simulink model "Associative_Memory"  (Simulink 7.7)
settings: Solver=ode113  StartTime=0.0  StopTime=20  RelTol=3e-14
undefined symbols (not defined in the file or in its folder): sigbuilder_block
libraries: fl_lib x51, nesl_utility x22, Memristor_lib x2

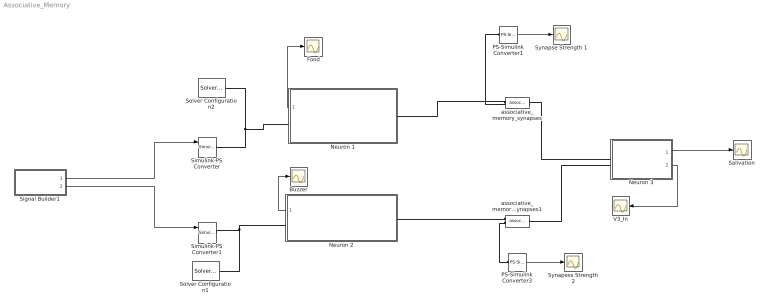
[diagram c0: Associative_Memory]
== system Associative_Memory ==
  Buzzer : Scope
  Food : Scope
  Neuron 1 : Subsystem
  Neuron 2 : Subsystem
  Neuron 3 : Subsystem
  PS-Simulink Converter1 : nesl_utility/PS-Simulink Converter  SystemSampleTime=-1  PhysicalDomain=network_engine_domain  LeftPortType=input  RightPortType=output  SubClassName=ps_output  Unit=1  AffineConversion=off
  PS-Simulink Converter3 : nesl_utility/PS-Simulink Converter  SystemSampleTime=-1  PhysicalDomain=network_engine_domain  LeftPortType=input  RightPortType=output  SubClassName=ps_output  Unit=1  AffineConversion=off
  Salivation : Scope
  Signal Builder1 : Subsystem  Tag=STV Subsys  LoadFcn=sigbuilder_block('load');  StartFcn=sigbuilder_block('start');  StopFcn=sigbuilder_block('stop');  ClipboardFcn=sigbuilder_block('clipboard');
  Simulink-PS Converter : nesl_utility/Simulink-PS Converter  SystemSampleTime=-1  PhysicalDomain=network_engine_domain  LeftPortType=input  RightPortType=output  SubClassName=ps_input  Unit=1  AffineConversion=off  InputFilterTimeConstant=.001  UdotUserProvided=2
  Simulink-PS Converter1 : nesl_utility/Simulink-PS Converter  SystemSampleTime=-1  PhysicalDomain=network_engine_domain  LeftPortType=input  RightPortType=output  SubClassName=ps_input  Unit=1  AffineConversion=off  InputFilterTimeConstant=.001  UdotUserProvided=2
  Solver Configuration1 : nesl_utility/Solver Configuration  SystemSampleTime=-1  PhysicalDomain=network_engine_domain  LeftPortType=input  RightPortType=generic  SubClassName=solver  Accelerate=off  Profile=off  ResidualTolerance=1e-9  MaxNonlinIter=3  MaxModeIter=2  DoFixedCost=off  UseLocalSampling=off  DoDC=off  LinearAlgebra=Sparse  LocalSolverSampleTime=.001  LocalSolverChoice=NE_BACKWARD_EULER_ADVANCER  UseLocalSolver=off
  Solver Configuration2 : nesl_utility/Solver Configuration  SystemSampleTime=-1  PhysicalDomain=network_engine_domain  LeftPortType=input  RightPortType=generic  SubClassName=solver  Accelerate=off  Profile=off  ResidualTolerance=1e-9  MaxNonlinIter=3  MaxModeIter=2  DoFixedCost=off  UseLocalSampling=off  DoDC=off  LinearAlgebra=Sparse  LocalSolverSampleTime=.001  LocalSolverChoice=NE_BACKWARD_EULER_ADVANCER  UseLocalSolver=off
  Synapse Strength 1 : Scope
  Synapses Strength 2 : Scope
  V3_In : Scope
  associative_memory_synapses : Memristor_lib/associative_memory_synapses  SystemSampleTime=-1  a=0 Ohm/s/V  B=15000 Ohm/s/V  VT=4 V  R1=675 Ohm  R2=1e+4 Ohm  x0=675 Ohm  i_Log=off  v_Log=off  x_Log=off  LocalVarNames=|i|v|x  LocalVarDescs=|i|v|x  LocalVarLogging=[0 0 0]
  associative_memory_synapses1 : Memristor_lib/associative_memory_synapses  SystemSampleTime=-1  a=0 Ohm/s/V  B=15000 Ohm/s/V  VT=4 V  R1=675 Ohm  R2=1e+4 Ohm  x0=1e+4 Ohm  i_Log=off  v_Log=off  x_Log=off  LocalVarNames=|i|v|x  LocalVarDescs=|i|v|x  LocalVarLogging=[0 0 0]
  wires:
  Signal Builder1/1(Food) -> Simulink-PS Converter/1
  Signal Builder1/2(Buzzer) -> Simulink-PS Converter1/1
  Neuron 3/1(Out1) -> Salivation/1
  PS-Simulink Converter3/1 -> Synapses Strength 2/1
  PS-Simulink Converter1/1 -> Synapse Strength 1/1
  Neuron 1/1(Input 1) -> Food/1
  Neuron 2/1(Input 2) -> Buzzer/1
  Neuron 3/2(V3_In) -> V3_In/1
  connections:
  Neuron 2/LConn1 -- associative_memory_synapses1/RConn1
  associative_memory_synapses/LConn1 -- Neuron 3/LConn1
  associative_memory_synapses1/LConn1 -- Neuron 3/LConn2
  PS-Simulink Converter1/LConn1 -- associative_memory_synapses/RConn2
  associative_memory_synapses/RConn1 -- Neuron 1/LConn1
  Solver Configuration2/RConn1 -- Simulink-PS Converter/RConn1 -- Neuron 1/RConn1
  Simulink-PS Converter1/RConn1 -- Neuron 2/RConn1 -- Solver Configuration1/RConn1
  associative_memory_synapses1/RConn2 -- PS-Simulink Converter3/LConn1

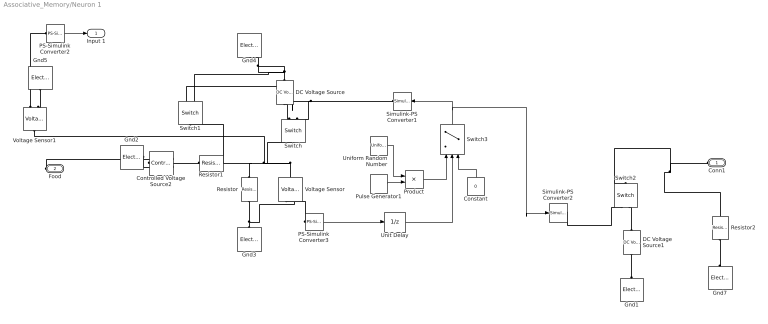
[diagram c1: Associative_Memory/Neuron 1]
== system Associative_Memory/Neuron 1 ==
  Constant : Constant  Value=0
  Controlled Voltage Source2 : fl_lib/Electrical/Electrical Sources/Controlled Voltage Source  SystemSampleTime=-1  i_Log=off  v_Log=off  LocalVarNames=|i|v  LocalVarDescs=|i|v  LocalVarLogging=[0 0]
  DC Voltage Source : fl_lib/Electrical/Electrical Sources/DC Voltage Source  SystemSampleTime=-1  v0=-2.5 V  i_Log=off  v_Log=off  LocalVarNames=|i|v  LocalVarDescs=|i|v  LocalVarLogging=[0 0]
  DC Voltage Source1 : fl_lib/Electrical/Electrical Sources/DC Voltage Source  SystemSampleTime=-1  v0=2.5 V  i_Log=off  v_Log=off  LocalVarNames=|i|v  LocalVarDescs=|i|v  LocalVarLogging=[0 0]
  Gnd{1..5,7} (6 alike) : fl_lib/Electrical/Electrical Elements/Electrical Reference  SystemSampleTime=-1  i_Log=off  LocalVarNames=|i  LocalVarDescs=|i  LocalVarLogging=0
  PS-Simulink Converter2 : nesl_utility/PS-Simulink Converter  SystemSampleTime=-1  PhysicalDomain=network_engine_domain  LeftPortType=input  RightPortType=output  SubClassName=ps_output  Unit=1  AffineConversion=off
  PS-Simulink Converter3 : nesl_utility/PS-Simulink Converter  SystemSampleTime=-1  PhysicalDomain=network_engine_domain  LeftPortType=input  RightPortType=output  SubClassName=ps_output  Unit=1  AffineConversion=off
  Product : Product  SampleTime=.001
  Pulse Generator1 : DiscretePulseGenerator  PulseType=Time based  Amplitude=1.1  Period=.1  PulseWidth=50
  Resistor : fl_lib/Electrical/Electrical Elements/Resistor  SystemSampleTime=-1  R=100 Ohm  i_Log=off  v_Log=off  LocalVarNames=|i|v  LocalVarDescs=|i|v  LocalVarLogging=[0 0]
  Resistor1 : fl_lib/Electrical/Electrical Elements/Resistor  SystemSampleTime=-1  R=50 Ohm  i_Log=off  v_Log=off  LocalVarNames=|i|v  LocalVarDescs=|i|v  LocalVarLogging=[0 0]
  Resistor2 : fl_lib/Electrical/Electrical Elements/Resistor  SystemSampleTime=-1  R=20000 Ohm  i_Log=off  v_Log=off  LocalVarNames=|i|v  LocalVarDescs=|i|v  LocalVarLogging=[0 0]
  Simulink-PS Converter1 : nesl_utility/Simulink-PS Converter  SystemSampleTime=-1  PhysicalDomain=network_engine_domain  LeftPortType=input  RightPortType=output  SubClassName=ps_input  Unit=1  AffineConversion=off  InputFilterTimeConstant=.001  UdotUserProvided=0
  Simulink-PS Converter2 : nesl_utility/Simulink-PS Converter  SystemSampleTime=-1  PhysicalDomain=network_engine_domain  LeftPortType=input  RightPortType=output  SubClassName=ps_input  Unit=1  AffineConversion=off  InputFilterTimeConstant=.001  UdotUserProvided=0
  Switch : fl_lib/Electrical/Electrical Elements/Switch  SystemSampleTime=-1  R_closed=0.01 Ohm  G_open=1e-8 1/Ohm  Threshold=.4  i_Log=off  v_Log=off  LocalVarNames=|i|v  LocalVarDescs=|i|v  LocalVarLogging=[0 0]
  Switch1 : fl_lib/Electrical/Electrical Elements/Switch  SystemSampleTime=-1  R_closed=0.01 Ohm  G_open=1e-8 1/Ohm  Threshold=1.5  i_Log=off  v_Log=off  LocalVarNames=|i|v  LocalVarDescs=|i|v  LocalVarLogging=[0 0]
  Switch2 : fl_lib/Electrical/Electrical Elements/Switch  SystemSampleTime=-1  R_closed=0.01 Ohm  G_open=1e-8 1/Ohm  Threshold=.4  i_Log=off  v_Log=off  LocalVarNames=|i|v  LocalVarDescs=|i|v  LocalVarLogging=[0 0]
  Switch3 : Switch  Threshold=1.5  SampleTime=.001
  Uniform Random Number : UniformRandomNumber  Minimum=0  Maximum=1.75  SampleTime=0.001
  Unit Delay : UnitDelay  SampleTime=.001
  Voltage Sensor : fl_lib/Electrical/Electrical Sensors/Voltage Sensor  SystemSampleTime=-1  i1_Log=off  v1_Log=off  LocalVarNames=|i1|v1  LocalVarDescs=|i1|v1  LocalVarLogging=[0 0]
  Voltage Sensor1 : fl_lib/Electrical/Electrical Sensors/Voltage Sensor  SystemSampleTime=-1  i1_Log=off  v1_Log=off  LocalVarNames=|i1|v1  LocalVarDescs=|i1|v1  LocalVarLogging=[0 0]
  Conn1 : PMIOPort  Port=1  Side=Left
  Food : PMIOPort  Port=2  Side=Right
  Input 1 : Outport
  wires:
  PS-Simulink Converter3/1 -> Unit Delay/1
  PS-Simulink Converter2/1 -> Input 1/1
  Pulse Generator1/1 -> Product/2
  Constant/1 -> Switch3/3
  Switch3/1 -> Simulink-PS Converter2/1, Simulink-PS Converter1/1
  Unit Delay/1 -> Switch3/2
  Uniform Random Number/1 -> Product/1
  Product/1 -> Switch3/1
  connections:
  Gnd2/LConn1 -- Controlled Voltage Source2/RConn2
  DC Voltage Source/LConn1 -- Switch/RConn2
  DC Voltage Source/RConn1 -- Gnd4/LConn1 -- Switch1/RConn2
  Gnd3/LConn1 -- Resistor/RConn1 -- Voltage Sensor/RConn2
  PS-Simulink Converter3/LConn1 -- Voltage Sensor/RConn1
  Voltage Sensor/LConn1 -- Switch/LConn1 -- Resistor/LConn1 -- Resistor1/LConn1 -- Voltage Sensor1/LConn1
  Simulink-PS Converter1/RConn1 -- Switch/RConn1 -- Switch1/RConn1
  Switch2/LConn1 -- Resistor2/LConn1 -- Conn1/RConn1
  Food/RConn1 -- Controlled Voltage Source2/RConn1
  Simulink-PS Converter2/RConn1 -- Switch2/RConn1
  DC Voltage Source1/LConn1 -- Switch2/RConn2
  DC Voltage Source1/RConn1 -- Gnd1/LConn1
  Gnd5/LConn1 -- Voltage Sensor1/RConn2
  Voltage Sensor1/RConn1 -- PS-Simulink Converter2/LConn1
  Resistor1/RConn1 -- Switch1/LConn1 -- Controlled Voltage Source2/LConn1
  Resistor2/RConn1 -- Gnd7/LConn1

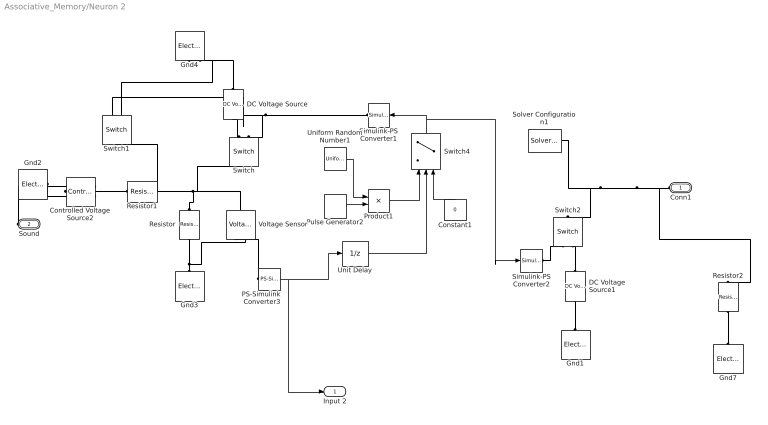
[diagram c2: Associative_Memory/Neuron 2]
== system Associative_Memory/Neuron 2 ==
  Constant1 : Constant  Value=0
  Controlled Voltage Source2 : fl_lib/Electrical/Electrical Sources/Controlled Voltage Source  SystemSampleTime=-1  i_Log=off  v_Log=off  LocalVarNames=|i|v  LocalVarDescs=|i|v  LocalVarLogging=[0 0]
  DC Voltage Source : fl_lib/Electrical/Electrical Sources/DC Voltage Source  SystemSampleTime=-1  v0=-2.5 V  i_Log=off  v_Log=off  LocalVarNames=|i|v  LocalVarDescs=|i|v  LocalVarLogging=[0 0]
  DC Voltage Source1 : fl_lib/Electrical/Electrical Sources/DC Voltage Source  SystemSampleTime=-1  v0=2.5 V  i_Log=off  v_Log=off  LocalVarNames=|i|v  LocalVarDescs=|i|v  LocalVarLogging=[0 0]
  Gnd{1..4,7} (5 alike) : fl_lib/Electrical/Electrical Elements/Electrical Reference  SystemSampleTime=-1  i_Log=off  LocalVarNames=|i  LocalVarDescs=|i  LocalVarLogging=0
  PS-Simulink Converter3 : nesl_utility/PS-Simulink Converter  SystemSampleTime=-1  PhysicalDomain=network_engine_domain  LeftPortType=input  RightPortType=output  SubClassName=ps_output  Unit=1  AffineConversion=off
  Product1 : Product  SampleTime=.001
  Pulse Generator2 : DiscretePulseGenerator  PulseType=Time based  Amplitude=1.1  Period=.1  PulseWidth=50
  Resistor : fl_lib/Electrical/Electrical Elements/Resistor  SystemSampleTime=-1  R=100 Ohm  i_Log=off  v_Log=off  LocalVarNames=|i|v  LocalVarDescs=|i|v  LocalVarLogging=[0 0]
  Resistor1 : fl_lib/Electrical/Electrical Elements/Resistor  SystemSampleTime=-1  R=50 Ohm  i_Log=off  v_Log=off  LocalVarNames=|i|v  LocalVarDescs=|i|v  LocalVarLogging=[0 0]
  Resistor2 : fl_lib/Electrical/Electrical Elements/Resistor  SystemSampleTime=-1  R=1 Ohm  i_Log=off  v_Log=off  LocalVarNames=|i|v  LocalVarDescs=|i|v  LocalVarLogging=[0 0]
  Simulink-PS Converter1 : nesl_utility/Simulink-PS Converter  SystemSampleTime=-1  PhysicalDomain=network_engine_domain  LeftPortType=input  RightPortType=output  SubClassName=ps_input  Unit=1  AffineConversion=off  InputFilterTimeConstant=.001  UdotUserProvided=0
  Simulink-PS Converter2 : nesl_utility/Simulink-PS Converter  SystemSampleTime=-1  PhysicalDomain=network_engine_domain  LeftPortType=input  RightPortType=output  SubClassName=ps_input  Unit=1  AffineConversion=off  InputFilterTimeConstant=.001  UdotUserProvided=0
  Solver Configuration1 : nesl_utility/Solver Configuration  SystemSampleTime=-1  PhysicalDomain=network_engine_domain  LeftPortType=input  RightPortType=generic  SubClassName=solver  Accelerate=off  Profile=off  ResidualTolerance=1e-9  MaxNonlinIter=3  MaxModeIter=2  DoFixedCost=off  UseLocalSampling=off  DoDC=off  LinearAlgebra=Sparse  LocalSolverSampleTime=.001  LocalSolverChoice=NE_BACKWARD_EULER_ADVANCER  UseLocalSolver=off
  Switch : fl_lib/Electrical/Electrical Elements/Switch  SystemSampleTime=-1  R_closed=0.01 Ohm  G_open=1e-8 1/Ohm  Threshold=.4  i_Log=off  v_Log=off  LocalVarNames=|i|v  LocalVarDescs=|i|v  LocalVarLogging=[0 0]
  Switch1 : fl_lib/Electrical/Electrical Elements/Switch  SystemSampleTime=-1  R_closed=0.01 Ohm  G_open=1e-8 1/Ohm  Threshold=1.5  i_Log=off  v_Log=off  LocalVarNames=|i|v  LocalVarDescs=|i|v  LocalVarLogging=[0 0]
  Switch2 : fl_lib/Electrical/Electrical Elements/Switch  SystemSampleTime=-1  R_closed=0.01 Ohm  G_open=1e-8 1/Ohm  Threshold=.4  i_Log=off  v_Log=off  LocalVarNames=|i|v  LocalVarDescs=|i|v  LocalVarLogging=[0 0]
  Switch4 : Switch  Threshold=1.5  SampleTime=.001
  Uniform Random Number1 : UniformRandomNumber  Minimum=0  Maximum=1.75  SampleTime=.001
  Unit Delay : UnitDelay  SampleTime=.001
  Voltage Sensor : fl_lib/Electrical/Electrical Sensors/Voltage Sensor  SystemSampleTime=-1  i1_Log=off  v1_Log=off  LocalVarNames=|i1|v1  LocalVarDescs=|i1|v1  LocalVarLogging=[0 0]
  Conn1 : PMIOPort  Port=1  Side=Left
  Sound : PMIOPort  Port=2  Side=Right
  Input 2 : Outport
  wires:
  PS-Simulink Converter3/1 -> Unit Delay/1, Input 2/1
  Switch4/1 -> Simulink-PS Converter1/1, Simulink-PS Converter2/1
  Pulse Generator2/1 -> Product1/2
  Constant1/1 -> Switch4/3
  Unit Delay/1 -> Switch4/2
  Uniform Random Number1/1 -> Product1/1
  Product1/1 -> Switch4/1
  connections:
  Resistor1/RConn1 -- Controlled Voltage Source2/LConn1 -- Switch1/LConn1
  Gnd2/LConn1 -- Controlled Voltage Source2/RConn2
  DC Voltage Source/LConn1 -- Switch/RConn2
  Gnd4/LConn1 -- DC Voltage Source/RConn1 -- Switch1/RConn2
  Gnd3/LConn1 -- Resistor/RConn1 -- Voltage Sensor/RConn2
  PS-Simulink Converter3/LConn1 -- Voltage Sensor/RConn1
  Resistor/LConn1 -- Voltage Sensor/LConn1 -- Switch/LConn1 -- Resistor1/LConn1
  Simulink-PS Converter1/RConn1 -- Switch/RConn1 -- Switch1/RConn1
  Conn1/RConn1 -- Switch2/LConn1 -- Solver Configuration1/RConn1 -- Resistor2/LConn1
  Sound/RConn1 -- Controlled Voltage Source2/RConn1
  DC Voltage Source1/LConn1 -- Switch2/RConn2
  DC Voltage Source1/RConn1 -- Gnd1/LConn1
  Resistor2/RConn1 -- Gnd7/LConn1
  Simulink-PS Converter2/RConn1 -- Switch2/RConn1

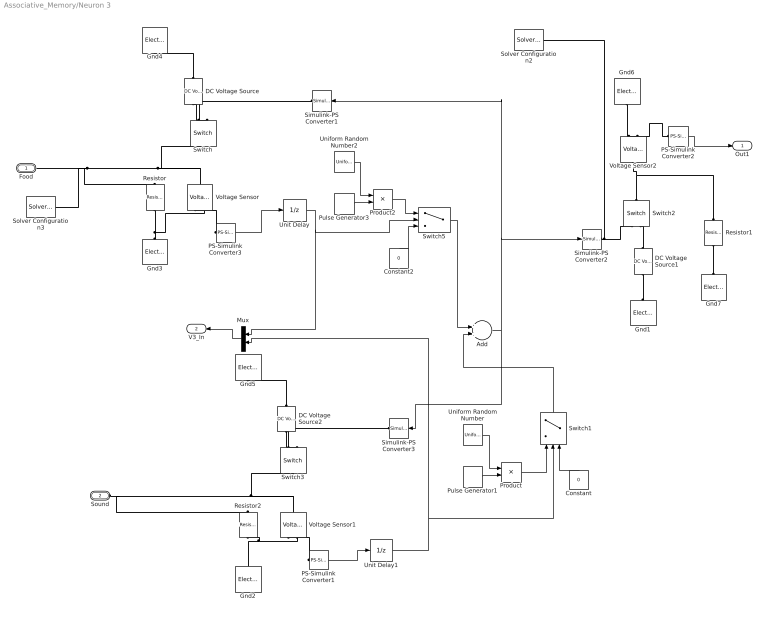
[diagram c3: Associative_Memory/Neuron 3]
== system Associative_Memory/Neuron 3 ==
  Add : Sum  SampleTime=.001
  Constant : Constant  Value=0
  Constant2 : Constant  Value=0
  DC Voltage Source : fl_lib/Electrical/Electrical Sources/DC Voltage Source  SystemSampleTime=-1  v0=-2.5 V  i_Log=off  v_Log=off  LocalVarNames=|i|v  LocalVarDescs=|i|v  LocalVarLogging=[0 0]
  DC Voltage Source1 : fl_lib/Electrical/Electrical Sources/DC Voltage Source  SystemSampleTime=-1  v0=2.5 V  i_Log=off  v_Log=off  LocalVarNames=|i|v  LocalVarDescs=|i|v  LocalVarLogging=[0 0]
  DC Voltage Source2 : fl_lib/Electrical/Electrical Sources/DC Voltage Source  SystemSampleTime=-1  v0=-2.5 V  i_Log=off  v_Log=off  LocalVarNames=|i|v  LocalVarDescs=|i|v  LocalVarLogging=[0 0]
  Gnd{1..7} (7 alike) : fl_lib/Electrical/Electrical Elements/Electrical Reference  SystemSampleTime=-1  i_Log=off  LocalVarNames=|i  LocalVarDescs=|i  LocalVarLogging=0
  Mux : Mux  Inputs=2
  PS-Simulink Converter1 : nesl_utility/PS-Simulink Converter  SystemSampleTime=-1  PhysicalDomain=network_engine_domain  LeftPortType=input  RightPortType=output  SubClassName=ps_output  Unit=1  AffineConversion=off
  PS-Simulink Converter2 : nesl_utility/PS-Simulink Converter  SystemSampleTime=-1  PhysicalDomain=network_engine_domain  LeftPortType=input  RightPortType=output  SubClassName=ps_output  Unit=1  AffineConversion=off
  PS-Simulink Converter3 : nesl_utility/PS-Simulink Converter  SystemSampleTime=-1  PhysicalDomain=network_engine_domain  LeftPortType=input  RightPortType=output  SubClassName=ps_output  Unit=1  AffineConversion=off
  Product : Product  SampleTime=.001
  Product2 : Product  SampleTime=.001
  Pulse Generator1 : DiscretePulseGenerator  PulseType=Time based  Amplitude=1.1  Period=.1  PulseWidth=50
  Pulse Generator3 : DiscretePulseGenerator  PulseType=Time based  Amplitude=1.1  Period=.1  PulseWidth=50
  Resistor : fl_lib/Electrical/Electrical Elements/Resistor  SystemSampleTime=-1  R=10000 Ohm  i_Log=off  v_Log=off  LocalVarNames=|i|v  LocalVarDescs=|i|v  LocalVarLogging=[0 0]
  Resistor1 : fl_lib/Electrical/Electrical Elements/Resistor  SystemSampleTime=-1  R=20000 Ohm  i_Log=off  v_Log=off  LocalVarNames=|i|v  LocalVarDescs=|i|v  LocalVarLogging=[0 0]
  Resistor2 : fl_lib/Electrical/Electrical Elements/Resistor  SystemSampleTime=-1  R=10000 Ohm  i_Log=off  v_Log=off  LocalVarNames=|i|v  LocalVarDescs=|i|v  LocalVarLogging=[0 0]
  Simulink-PS Converter1 : nesl_utility/Simulink-PS Converter  SystemSampleTime=-1  PhysicalDomain=network_engine_domain  LeftPortType=input  RightPortType=output  SubClassName=ps_input  Unit=1  AffineConversion=off  InputFilterTimeConstant=.001  UdotUserProvided=0
  Simulink-PS Converter2 : nesl_utility/Simulink-PS Converter  SystemSampleTime=-1  PhysicalDomain=network_engine_domain  LeftPortType=input  RightPortType=output  SubClassName=ps_input  Unit=1  AffineConversion=off  InputFilterTimeConstant=.001  UdotUserProvided=0
  Simulink-PS Converter3 : nesl_utility/Simulink-PS Converter  SystemSampleTime=-1  PhysicalDomain=network_engine_domain  LeftPortType=input  RightPortType=output  SubClassName=ps_input  Unit=1  AffineConversion=off  InputFilterTimeConstant=.001  UdotUserProvided=0
  Solver Configuration2 : nesl_utility/Solver Configuration  SystemSampleTime=-1  PhysicalDomain=network_engine_domain  LeftPortType=input  RightPortType=generic  SubClassName=solver  Accelerate=off  Profile=off  ResidualTolerance=1e-9  MaxNonlinIter=3  MaxModeIter=2  DoFixedCost=off  UseLocalSampling=off  DoDC=off  LinearAlgebra=Sparse  LocalSolverSampleTime=.001  LocalSolverChoice=NE_BACKWARD_EULER_ADVANCER  UseLocalSolver=off
  Solver Configuration3 : nesl_utility/Solver Configuration  SystemSampleTime=-1  PhysicalDomain=network_engine_domain  LeftPortType=input  RightPortType=generic  SubClassName=solver  Accelerate=off  Profile=off  ResidualTolerance=1e-9  MaxNonlinIter=3  MaxModeIter=2  DoFixedCost=off  UseLocalSampling=off  DoDC=off  LinearAlgebra=Sparse  LocalSolverSampleTime=.001  LocalSolverChoice=NE_BACKWARD_EULER_ADVANCER  UseLocalSolver=off
  Switch : fl_lib/Electrical/Electrical Elements/Switch  SystemSampleTime=-1  R_closed=0.01 Ohm  G_open=1e-8 1/Ohm  Threshold=.4  i_Log=off  v_Log=off  LocalVarNames=|i|v  LocalVarDescs=|i|v  LocalVarLogging=[0 0]
  Switch1 : Switch  Threshold=1.5  SampleTime=.001
  Switch2 : fl_lib/Electrical/Electrical Elements/Switch  SystemSampleTime=-1  R_closed=0.01 Ohm  G_open=1e-8 1/Ohm  Threshold=.4  i_Log=off  v_Log=off  LocalVarNames=|i|v  LocalVarDescs=|i|v  LocalVarLogging=[0 0]
  Switch3 : fl_lib/Electrical/Electrical Elements/Switch  SystemSampleTime=-1  R_closed=0.01 Ohm  G_open=1e-8 1/Ohm  Threshold=.4  i_Log=off  v_Log=off  LocalVarNames=|i|v  LocalVarDescs=|i|v  LocalVarLogging=[0 0]
  Switch5 : Switch  Threshold=1.5  SampleTime=.001
  Uniform Random Number : UniformRandomNumber  Minimum=0  Maximum=1.75  SampleTime=.001
  Uniform Random Number2 : UniformRandomNumber  Minimum=0  Maximum=1.75  SampleTime=.001
  Unit Delay : UnitDelay  SampleTime=.01
  Unit Delay1 : UnitDelay  SampleTime=.01
  Voltage Sensor : fl_lib/Electrical/Electrical Sensors/Voltage Sensor  SystemSampleTime=-1  i1_Log=off  v1_Log=off  LocalVarNames=|i1|v1  LocalVarDescs=|i1|v1  LocalVarLogging=[0 0]
  Voltage Sensor1 : fl_lib/Electrical/Electrical Sensors/Voltage Sensor  SystemSampleTime=-1  i1_Log=off  v1_Log=off  LocalVarNames=|i1|v1  LocalVarDescs=|i1|v1  LocalVarLogging=[0 0]
  Voltage Sensor2 : fl_lib/Electrical/Electrical Sensors/Voltage Sensor  SystemSampleTime=-1  i1_Log=off  v1_Log=off  LocalVarNames=|i1|v1  LocalVarDescs=|i1|v1  LocalVarLogging=[0 0]
  Food : PMIOPort  Port=1  Side=Left
  Sound : PMIOPort  Port=2  Side=Left
  Out1 : Outport
  V3_In : Outport  Port=2
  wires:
  PS-Simulink Converter3/1 -> Unit Delay/1
  PS-Simulink Converter1/1 -> Unit Delay1/1
  Add/1 -> Simulink-PS Converter1/1, Simulink-PS Converter2/1, Simulink-PS Converter3/1
  PS-Simulink Converter2/1 -> Out1/1
  Unit Delay/1 -> Mux/1, Switch5/2
  Unit Delay1/1 -> Mux/2, Switch1/2
  Mux/1 -> V3_In/1
  Pulse Generator3/1 -> Product2/2
  Constant2/1 -> Switch5/3
  Uniform Random Number2/1 -> Product2/1
  Product2/1 -> Switch5/1
  Switch5/1 -> Add/1
  Pulse Generator1/1 -> Product/2
  Constant/1 -> Switch1/3
  Uniform Random Number/1 -> Product/1
  Product/1 -> Switch1/1
  Switch1/1 -> Add/2
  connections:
  DC Voltage Source/LConn1 -- Switch/RConn2
  DC Voltage Source/RConn1 -- Gnd4/LConn1
  Gnd3/LConn1 -- Resistor/RConn1 -- Voltage Sensor/RConn2
  PS-Simulink Converter3/LConn1 -- Voltage Sensor/RConn1
  Switch/RConn1 -- Simulink-PS Converter1/RConn1
  Voltage Sensor/LConn1 -- Switch/LConn1 -- Resistor/LConn1 -- Food/RConn1 -- Solver Configuration3/RConn1
  Simulink-PS Converter2/RConn1 -- Switch2/RConn1 -- Solver Configuration2/RConn1
  DC Voltage Source1/LConn1 -- Switch2/RConn2
  DC Voltage Source1/RConn1 -- Gnd1/LConn1
  DC Voltage Source2/RConn1 -- Gnd5/LConn1
  Voltage Sensor1/RConn2 -- Gnd2/LConn1 -- Resistor2/RConn1
  Sound/RConn1 -- Switch3/LConn1 -- Voltage Sensor1/LConn1 -- Resistor2/LConn1
  Switch3/RConn1 -- Simulink-PS Converter3/RConn1
  DC Voltage Source2/LConn1 -- Switch3/RConn2
  PS-Simulink Converter1/LConn1 -- Voltage Sensor1/RConn1
  Voltage Sensor2/LConn1 -- Switch2/LConn1 -- Resistor1/LConn1
  PS-Simulink Converter2/LConn1 -- Voltage Sensor2/RConn1
  Gnd6/LConn1 -- Voltage Sensor2/RConn2
  Resistor1/RConn1 -- Gnd7/LConn1

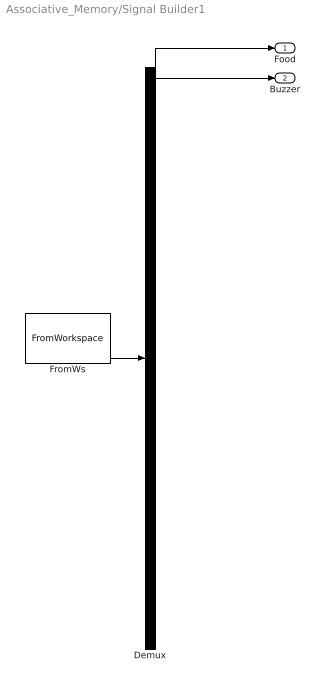
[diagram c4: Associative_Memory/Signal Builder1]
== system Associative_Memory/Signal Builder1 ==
  Demux : Demux  Tag=STV Demux  Outputs=2
  FromWs : FromWorkspace  Tag=STV FromWs  VariableName=tuvar  SampleTime=0  SigBuilderData=DataTag0  VnvData=DataTag1
  Food : Outport  Tag=STV Outport
  Buzzer : Outport  Tag=STV Outport  Port=2
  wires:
  FromWs/1 -> Demux/1
  Demux/1 -> Food/1
  Demux/2 -> Buzzer/1
